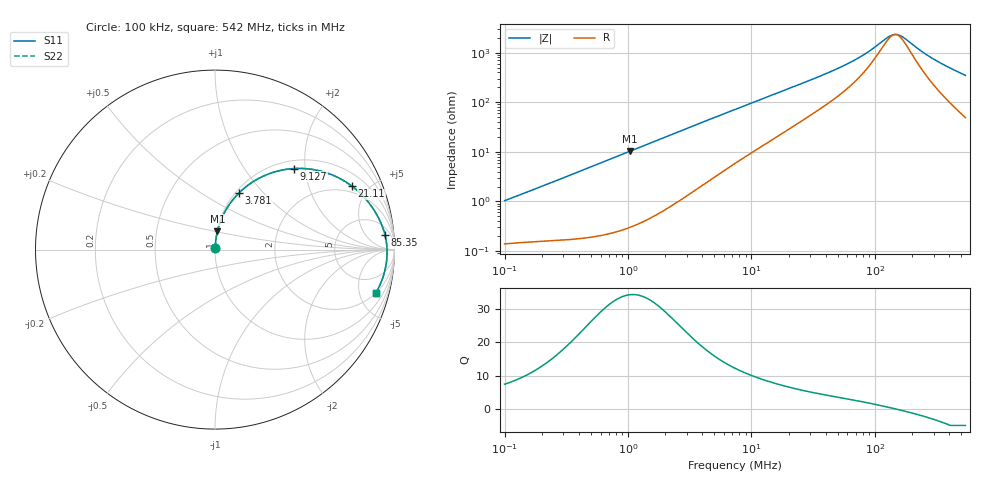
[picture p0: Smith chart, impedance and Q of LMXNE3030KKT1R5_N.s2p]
! LMXNE3030KKT1R5_N  S-PARAMETER MODEL  ( General Type )
! Model Generated by TAIYO YUDEN Corporation (https://www.yuden.co.jp/en/)
! Version 1.0
! TAIYO YUDEN Control No. 191023NI43SB-FBB
! Copyright(c) 2019 TAIYO YUDEN CO.,LTD. All Rights Reserved.
! Product Description (link to TY-COMPAS)
! https://ds.yuden.co.jp/TYCOMPAS/or/detail?pn=LMXNE3030KKT1R5NN&u=M
! Products Name : Inductors
! Characteristics :
!  Inductance : 1.5 uH , SRF(min) : 99 MHz , DC Resistance(max) : 0.09 Ohm
!  Rated Current : Saturation :1440 mA , Temp Rise : 1370 mA (40 degC)
!  Case Size : 3.0 x 3.0 / 0.118 x 0.118 [mm/inch] , Thickness : 1 / 0.039 [mm/inch]
!  (Conditions: Temperature = 25 degC , DC Bias Current/Voltage = 0A / 0V)
! External Node Assignments :
!  1  o---GGG---o  2
! GND o---------o GND
! Frequency Range : 0.1MHz  -  542.002916MHz  [ 402 STEP ]
# MHz S RI R 50
! Freq[MHz].  S11 Real  S11 Imag  S21 Real  S21 Imag  S12 Real  S12 Imag  S22 Real  S22 Imag
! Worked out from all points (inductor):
!   401 points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, 100 kHz to 542 MHz, reference 50 ohm
!   read as one part in series: L = 1.62 uH near 104.4 kHz
!   highest Q = 34.3 at 1.041 MHz (marker M1), where L = 1.58 uH
!   self-resonance near 145.8 MHz
!   S11 on the Smith chart (normalised r, x): 100 kHz: 1.00, +0.02; 3.781 MHz: 1.04, +0.74; 9.127 MHz: 1.17, +1.75; 21.11 MHz: 1.62, +3.90; 85.35 MHz: 10, +17; 542 MHz: 1.98, -6.90
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0.1  0.0015 0.0103  0.9985 -0.0103  0.9985 -0.0103  0.0015 0.0103
0.422129  0.00356 0.0419  0.9964 -0.0419  0.9964 -0.0419  0.00356 0.0419
1.041155  0.0135 0.1019  0.9865 -0.1019  0.9865 -0.1019  0.0135 0.1019
1.78193  0.0356 0.1697  0.9644 -0.1697  0.9644 -0.1697  0.0356 0.1697
2.680746  0.0745 0.243  0.9255 -0.243  0.9255 -0.243  0.0745 0.243
3.781078  0.1344 0.3163  0.8656 -0.3163  0.8656 -0.3163  0.1344 0.3163
5.219642  0.222 0.3844  0.778 -0.3844  0.778 -0.3844  0.222 0.3844
7.362085  0.3496 0.4375  0.6504 -0.4375  0.6504 -0.4375  0.3496 0.4375
9.127479  0.4415 0.4517  0.5585 -0.4517  0.5585 -0.4517  0.4415 0.4517
13.43943  0.6074 0.4322  0.3926 -0.4322  0.3926 -0.4322  0.6074 0.4322
21.10649  0.7628 0.3535  0.2372 -0.3535  0.2372 -0.3535  0.7628 0.3535
31.0775  0.85 0.2697  0.15 -0.2697  0.15 -0.2697  0.85 0.2697
55.52534  0.9218 0.1543  0.0782 -0.1543  0.0782 -0.1543  0.9218 0.1543
70.33577  0.9379 0.1132  0.0621 -0.1132  0.0621 -0.1132  0.9379 0.1132
85.34759  0.9471 0.0817  0.0529 -0.0817  0.0529 -0.0817  0.9471 0.0817
131.1872  0.9578 0.0159  0.0422 -0.0159  0.0422 -0.0159  0.9578 0.0159
146.0718  0.9587 -0.000249  0.0413 0.000249  0.0413 0.000249  0.9587 -0.000249
162.6453  0.9589 -0.0165  0.0411 0.0165  0.0411 0.0165  0.9589 -0.0165
239.4812  0.9541 -0.0778  0.0459 0.0778  0.0459 0.0778  0.9541 -0.0778
290.5939  0.9476 -0.1116  0.0524 0.1116  0.0524 0.1116  0.9476 -0.1116
401.1544  0.928 -0.1753  0.072 0.1753  0.072 0.1753  0.928 -0.1753
542.0029  0.8946 -0.2443  0.1054 0.2443  0.1054 0.2443  0.8946 -0.2443
